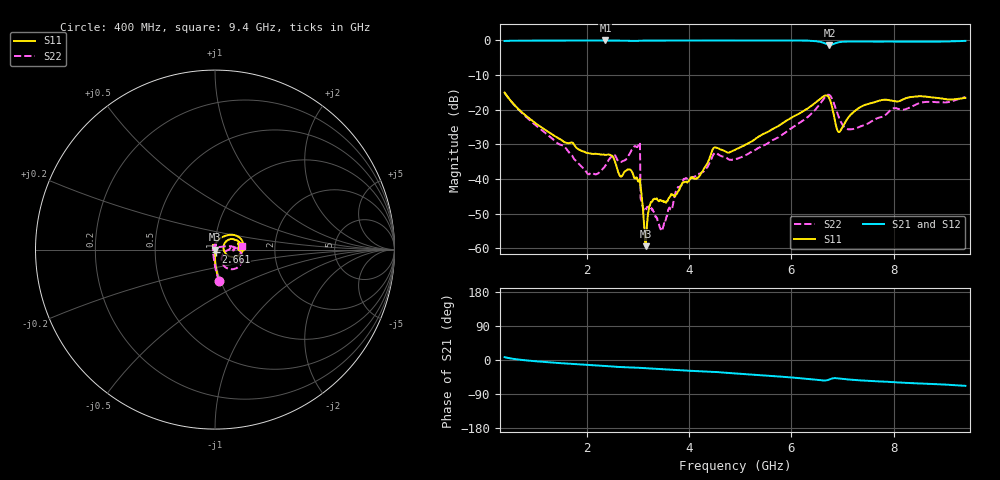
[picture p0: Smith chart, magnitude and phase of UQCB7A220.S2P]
!  Part Number  UQCB7A220  Mounting Orientation: Vertical
!  Description: RF capacitors
!  Application: Coupling, Bypass, Tuning, DC Block
!  Filters, Matching
# GHZ S DB R 50
! Freq  |S11|  S11 Ph  |S21|  S21 Ph  |S12|  S12 Ph  |S22|  S22 Ph
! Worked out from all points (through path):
!   801 points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, 400 MHz to 9.4 GHz, reference 50 ohm
!   highest |S21| = 0.00 dB at 2.369 GHz (marker M1); lowest = -1.3 dB at 6.745 GHz (marker M2)
!   group delay of S21, straight-line fit = 21.8 ps
!   lowest |S11| = -59.3 dB at 3.156 GHz (marker M3), VSWR 1.00, Z = 50 - j0.108 ohm
!   |S11| at or under -10 dB: start of sweep to end of sweep
!   |S22| runs from -54.7 to -15.1 dB; largest |S21 - S12| = 0.0012
!   S11 on the Smith chart (normalised r, x): 400 MHz: 0.99, -0.36; 2.661 GHz: 1.01, -0.02; 9.4 GHz: 1.35, +0.04
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0.4  -15.04 -82.0  -0.15 7.4  -0.15 7.4  -15.08 -82.6
1.908  -31.88 -85.0  -0.03 -11.9  -0.03 -11.9  -36.44 -133.4
2.178  -32.68 -76.9  -0.02 -14.2  -0.02 -14.2  -38.63 179.4
2.369  -32.99 -77.3  0.00 -15.8  -0.01 -15.8  -36.11 136.9
2.515  -33.54 -89.4  -0.01 -17.3  -0.01 -17.3  -33.03 102.2
2.661  -39.18 -75.2  -0.06 -18.6  -0.07 -18.6  -35.10 84.3
2.999  -40.39 -36.4  -0.12 -20.4  -0.12 -20.4  -30.63 86.0
3.1  -48.24 -158.2  -0.06 -21.2  -0.06 -21.2  -48.01 13.0
3.156  -59.34 -90.2  -0.05 -21.7  -0.05 -21.7  -48.55 13.0
3.269  -46.58 -80.5  -0.04 -22.6  -0.05 -22.6  -48.33 -47.5
3.404  -46.28 -116.0  -0.02 -23.7  -0.02 -23.7  -52.54 -153.3
3.494  -46.25 -135.6  -0.02 -24.5  -0.02 -24.5  -53.87 -156.2
3.91  -40.91 141.2  -0.04 -27.6  -0.04 -27.7  -40.02 160.0
4.18  -39.52 125.2  -0.02 -29.6  -0.02 -29.6  -38.51 129.3
4.495  -30.89 107.5  -0.01 -31.5  -0.02 -31.5  -32.58 94.3
4.9  -31.57 83.4  -0.01 -35.3  -0.01 -35.3  -34.24 43.2
6.408  -18.68 45.3  -0.12 -50.9  -0.12 -51.0  -20.91 11.8
6.745  -16.79 -9.5  -1.29 -51.4  -1.29 -51.4  -15.75 -34.6
6.936  -26.41 9.4  -0.50 -48.8  -0.50 -48.8  -22.48 -60.4
7.173  -21.23 36.6  -0.30 -52.1  -0.30 -52.1  -25.62 -29.3
7.904  -17.21 14.2  -0.31 -57.8  -0.31 -57.8  -20.55 5.5
9.4  -16.57 6.3  -0.12 -68.2  -0.12 -68.2  -16.32 8.5
